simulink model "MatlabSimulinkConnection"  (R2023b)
settings: Solver=VariableStepAuto  StartTime=0.0  StopTime=simTime  RelTol=1e-3
libraries: simulink x1

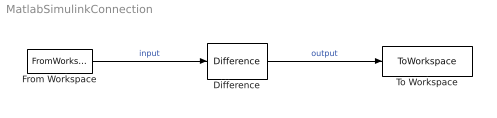
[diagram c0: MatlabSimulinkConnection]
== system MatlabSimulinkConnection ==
  Difference : simulink/Discrete/Difference  ICPrevInput=0.0  OutMin=[]  OutMax=[]  OutDataType=fixdt(1, 16)  OutScaling=2^-10  DoSatur=off
  From Workspace : FromWorkspace  VariableName=simIn
  To Workspace : ToWorkspace  VariableName=simOut  SampleTime=-1
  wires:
  Difference/1 -> To Workspace/1  "output"
  From Workspace/1 -> Difference/1  "input"
